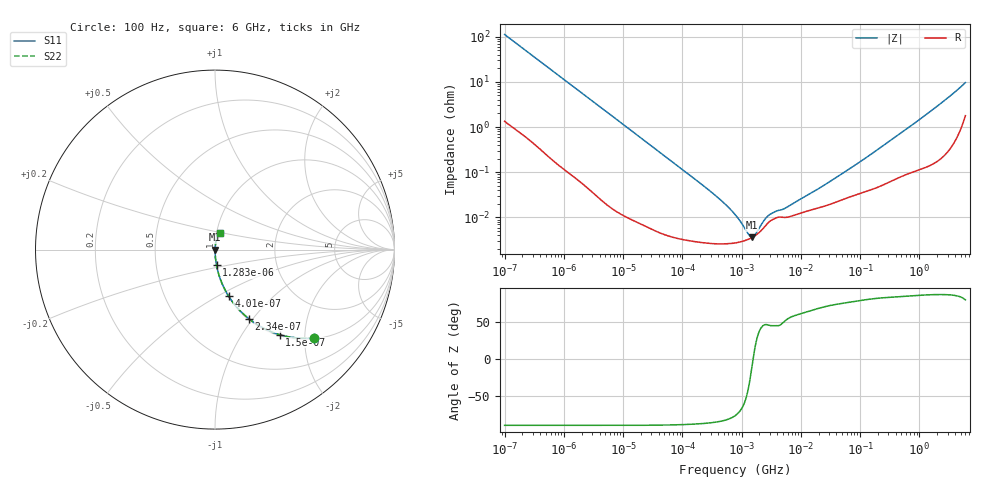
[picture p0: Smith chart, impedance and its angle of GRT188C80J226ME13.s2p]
!Murata Part Number: GRT188C80J226ME13
!These Parameters are Measured in Series Mode Connection
!Data Generated on Jun 19, 2026
!  o--ll--o
!Port1  Port2
!  o------o
!Operation Temp=25[degC], DC Bias Voltage=0[V]
!Freq. Start=100[Hz] Stop=6[GHz] 401[Steps]
# Hz S RI R 50
!Freq.(Hz) S11(Real) S11(Imag) S21(Real) S21(Imag) S12(Real) S12(Imag) S22(Real) S22(Imag)
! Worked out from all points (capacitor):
!   401 points, 100 Hz to 6 GHz, reference 50 ohm
!   read as one part in series: C = 14.2 uF near 109 Hz
!   lowest |Z| = 3.66 mohm at 1.516 MHz (marker M1)
!   series resonance near 1.565 MHz, so ESL is about 730 pH
!   S11 on the Smith chart (normalised r, x): 100 Hz: 1.03, -2.23; 150 Hz: 1.02, -1.49; 234 Hz: 1.01, -0.96; 401 Hz: 1.01, -0.56; 1.283 kHz: 1.00, -0.18; 6 GHz: 1.04, +0.19
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100  0.5533 -0.4912  0.4467 0.4912  0.4467 0.4912  0.5533 -0.4912
150  0.3597 -0.4739  0.6403 0.4739  0.6403 0.4739  0.3597 -0.4739
234  0.1896 -0.386  0.8104 0.386  0.8104 0.386  0.1896 -0.386
401  0.0758 -0.2591  0.9242 0.2591  0.9242 0.2591  0.0758 -0.2591
717  0.0258 -0.1534  0.9742 0.1534  0.9742 0.1534  0.0258 -0.1534
1283  0.00864 -0.0876  0.9914 0.0876  0.9914 0.0876  0.00864 -0.0876
2008  0.00377 -0.0564  0.9962 0.0564  0.9962 0.0564  0.00377 -0.0564
6433  0.000476 -0.0178  0.9995 0.0178  0.9995 0.0178  0.000476 -0.0178
40335  5.47e-05 -0.00286  0.9999 0.00286  0.9999 0.00286  5.47e-05 -0.00286
330837  2.65e-05 -0.000337  1 0.000337  1 0.000337  2.65e-05 -0.000337
541393  2.62e-05 -0.00019  1 0.00019  1 0.00019  2.62e-05 -0.00019
774597  2.74e-05 -0.000114  1 0.000114  1 0.000114  2.74e-05 -0.000114
926525  2.86e-05 -8.18e-05  1 8.18e-05  1 8.18e-05  2.86e-05 -8.18e-05
1516199  3.63e-05 -4.6e-06  1 4.6e-06  1 4.6e-06  3.63e-05 -4.6e-06
2594782  6.8e-05 7.09e-05  0.9999 -7.09e-05  0.9999 -7.09e-05  6.8e-05 7.09e-05
3712478  9.62e-05 9.54e-05  0.9999 -9.54e-05  0.9999 -9.54e-05  9.62e-05 9.54e-05
5554849  0.0001 0.000128  0.9999 -0.000128  0.9999 -0.000128  0.0001 0.000128
1.555665e7  0.000149 0.000326  0.9999 -0.000326  0.9999 -0.000326  0.000149 0.000326
7.797396e7  0.000306 0.00133  0.9997 -0.00133  0.9997 -0.00133  0.000306 0.00133
3.124326e8  0.00063 0.00481  0.9994 -0.00481  0.9994 -0.00481  0.00063 0.00481
1.95892e9  0.00249 0.0281  0.9975 -0.0281  0.9975 -0.0281  0.00249 0.0281
6e9  0.0259 0.0905  0.9741 -0.0905  0.9741 -0.0905  0.0259 0.0905
